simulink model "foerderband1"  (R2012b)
settings: Solver=ode45  StartTime=0.0  StopTime=20  MaxStep=0.01  RelTol=1e-3
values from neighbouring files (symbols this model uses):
  g = 9.89    [foerd_gleit_1.m]    (also in foerder_haft_gleit_1.m; foerder_haft_gleit_2.m; foerderband_1.m; position_reg_1.m)
  mu = m2/m1    (= 0.05)    [feder_masse_1.m]    (also in feder_masse_13.m; feder_masse_14.m; foerd_gleit_1.m = 0.9; foerder_haft_gleit_1.m = 0.5)
libraries: simulink x1

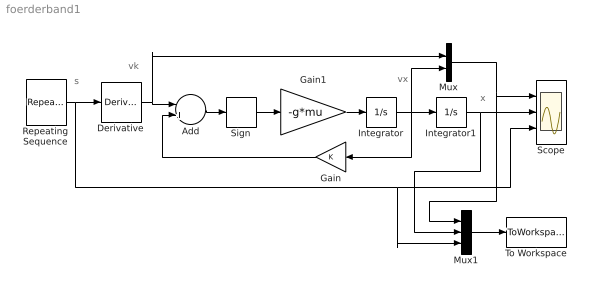
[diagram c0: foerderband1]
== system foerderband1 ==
  note: s
  note: x
  note: vk
  note: vx
  Add : Sum  Inputs=-+
  Derivative : Derivative
  Gain : Gain
  Gain1 : Gain  Gain=-g*mu
  Integrator : Integrator
  Integrator1 : Integrator
  Mux : Mux  Inputs=2
  Mux1 : Mux  Inputs=3
  Repeating Sequence : simulink/Sources/Repeating Sequence  rep_seq_t=tanr  rep_seq_y=s_anr
  Scope : Scope  NumInputPorts=3
  Sign : Signum  ZeroCross=off
  To Workspace : ToWorkspace  VariableName=y  SampleTime=-1  SaveFormat=Structure With Time
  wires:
  Add/1 -> Sign/1
  Integrator/1 -> Integrator1/1, Gain/1, Mux/2
  Gain/1 -> Add/2
  Sign/1 -> Gain1/1
  Gain1/1 -> Integrator/1
  Repeating Sequence/1 -> Mux1/3, Scope/3, Derivative/1
  Derivative/1 -> Mux/1, Add/1
  Mux1/1 -> To Workspace/1
  Mux/1 -> Mux1/1, Scope/1
  Integrator1/1 -> Mux1/2, Scope/2
